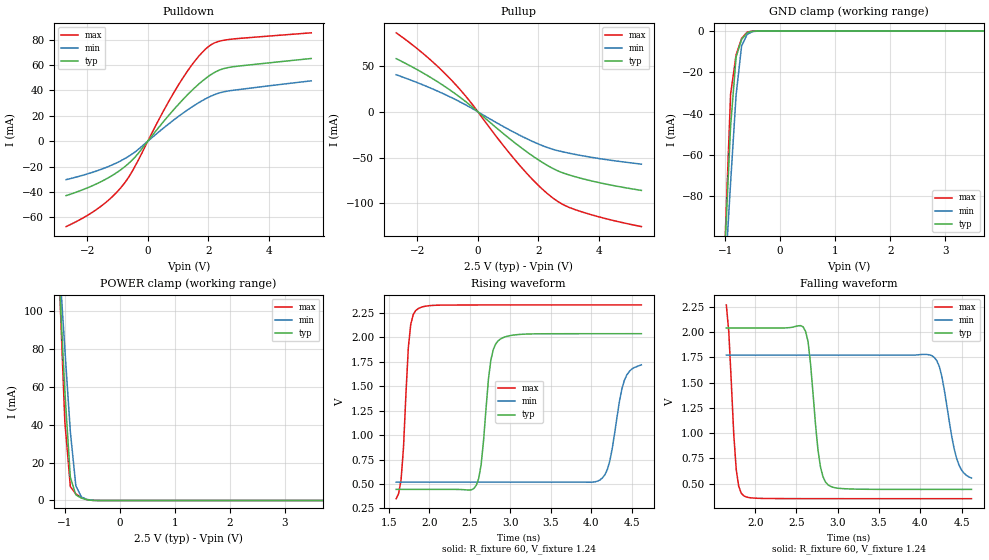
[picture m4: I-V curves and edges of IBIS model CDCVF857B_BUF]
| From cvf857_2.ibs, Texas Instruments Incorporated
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|   Diff. Driver Output  MODEL updated 8/2003
[Model]   CDCVF857B_BUF
Model_type   3-state
Polarity   Non-Inverting
| Signals   FBOUT,FBOUT-,Y0,Y0-, Y1,Y1-, Y2,Y2-, Y3,Y3-, Y4,Y4-,
|   Y5,Y5-, Y6,Y6-, Y7,Y7-, Y8,Y8-, Y9,Y9-
Vmeas = 1.25V   |Vref for timing measurements (crosspoint)
Cref = 14pF   |load capacitance for timing spec (to ground!)
Rref = 60   |60 Ohm to VDD/2 for timing measurements
Vref = 1.25V   |Timing specification test load voltage
| variable   typ   min   max
C_comp   2.4pF   2.0pF   2.7pF
[Temperature Range]   40.0   105   0
[Voltage range]   2.5V   2.3V   2.7V
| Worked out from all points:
|   slope of the pulldown table from 0 to 0.375 V, typ, clamps not added: 33.3 ohm
|   slope of the pullup table from 0 to 0.375 V, typ, clamps not added: 34.6 ohm
|   GND clamp passes 1 mA (typ) near -0.61 V on its own axis
|   POWER clamp passes 1 mA (typ) near -0.67 V on its own axis
|   rising waveform, R_fixture 60, V_fixture 1.24: 20-80 % time 105ps typ, 146ps min, 76.2ps max; typ from 0.444 V to 2.04 V
|   falling waveform, R_fixture 60, V_fixture 1.24: 20-80 % time 108ps typ, 157ps min, 74.9ps max; typ from 2.04 V to 0.445 V
[Pullup]
|   40C:2.5V:nominal 105C:2.3V:weak   0C:2.7V:strong
|   Voltage   I(typ)   I(min)   I(max)
-2.7V     58.06mA    40.49mA    86.29mA
-1.7V     40.25mA    27.85mA    60.54mA
-900mV    23.3mA     15.98mA    35.5mA
-300mV    8.384mA    5.704mA    12.94mA
700mV     -19.95mA   -13.47mA   -30.93mA
1.3V      -35.9mA    -24.18mA   -55.38mA
1.9V      -50.31mA   -33.72mA   -77.12mA
2.4V      -60.47mA   -40.15mA   -92.13mA
2.8V      -66.59mA   -43.63mA   -101mA
3.3V      -71.64mA   -47.04mA   -107.8mA
4.2V      -78.68mA   -51.97mA   -116.4mA
5.4V      -85.8mA    -57.13mA   -125.3mA
[Pulldown]
|   40C:2.5V:nominal   105C:2.3V:weak   0C:2.7V:strong
|   Voltage   I(typ)   I(min)   I(max)
-2.7V     -42.96mA   -30.37mA   -67.38mA
-1.6V     -32.59mA   -22.72mA   -52.28mA
-1.2V     -27.42mA   -18.96mA   -44.42mA
-800mV    -20.89mA   -14.29mA   -34.01mA
-400mV    -12.02mA   -8.101mA   -18.78mA
500mV     14.9mA     9.979mA    23.08mA
1.1V      31.31mA    21.04mA    47.7mA
1.5V      41.03mA    27.64mA    61.59mA
2V        51.1mA     34.55mA    74.57mA
2.3V      55.4mA     37.56mA    78.41mA
2.7V      58.27mA    39.76mA    80.29mA
5.4V      65.21mA    47.59mA    85.47mA
[GND Clamp]
|   40C:2.5V:nominal  105C:2.3V:weak   0C:2.7V:strong
|  Voltage   I(typ)   I(min)   I(max)
-2.7V     -1.103A    -887.8mA   -1.395A
-1.1V     -162.1mA   -163.9mA   -171.8mA
-900mV    -46.23mA   -73.5mA    -30.7mA
-800mV    -12.6mA    -30.96mA   -11.52mA
-700mV    -4.108mA   -7.28mA    -3.616mA
-600mV    -807.7uA   -1.647mA   -496.6uA
-500mV    -81.09uA   -268.7uA   -30.08uA
-300mV    -219.6nA   -2.842uA   -15.58nA
5.4V      252.8pA    5.148nA    125.2pA
[POWER Clamp]
|   40C:2.5V:nominal   105C:2.3V:weak   0C:2.7V:strong
|  Voltage   I(typ)   I(min)   I(max)
-2.7V     1.057A     849.3mA    1.339A
-1.1V     116.1mA    125.3mA    115.7mA
-1V       57.76mA    80.13mA    41.69mA
-900mV    12.21mA    36.35mA    7.299mA
-800mV    2.976mA    7.713mA    3.48mA
-700mV    1.27mA     1.885mA    1.613mA
-600mV    407.8uA    568.5uA    461.4uA
-400mV    5.905uA    16.46uA    4.279uA
5.4V      0A         0A         0A
[ramp]
| variable   typ   min   max
dV/dt_r   0.9566/1.0240E-10   0.7468/1.5201E-10   1.1331/6.9055E-11
dV/dt_f   0.9566/1.0535E-10   0.7468/1.6224E-10   1.1331/6.9424E-11
[Rising Waveform]
R_fixture = 60
V_fixture = 1.24
V_fixture_min = 1.14
V_fixture_max = 1.39
|   NOTE: WARNINGS generated by Innoveda Visual IBIS Editor are a best
|   compromise for ramp resulution and TPD prepresentation within
|   the 100 data point limits.
|   If rise/fall time analysis is mor important then TPD, use the
|   PLL-TYPE model which has better timing resolution.
|   40C:2.5V:nominal  105C:2.3V:weak   0C:2.7V:strong
|   Time   V(typ)   V(min)   V(max)
1.59ns    443.9mV    518mV      348.7mV
1.65ns    443.9mV    518mV      541.5mV
1.77ns    443.9mV    518mV      2.135V
1.86ns    443.9mV    518mV      2.294V
2.58ns    487.3mV    518mV      2.332V
2.76ns    1.768V     518mV      2.332V
2.85ns    1.966V     518mV      2.332V
4.11ns    2.038V     541.6mV    2.333V
4.41ns    2.038V     1.56V      2.333V
4.62ns    2.038V     1.719V     2.333V
[Falling Waveform]
R_fixture = 60
V_fixture = 1.24
V_fixture_min = 1.14
V_fixture_max = 1.39
|   40C:2.5V:nominal   105C:2.3V:weak  0C:2.7V:strong
|   Time   V(typ)   V(min)   V(max)
1.65ns    2.039V     1.77V      2.267V
1.77ns    2.039V     1.77V      640.7mV
1.86ns    2.039V     1.77V      382.1mV
2.61ns    2.006V     1.77V      353.6mV
2.76ns    836.2mV    1.77V      353.5mV
2.88ns    491.1mV    1.77V      353.4mV
4.14ns    444.7mV    1.765V     353.1mV
4.26ns    444.7mV    1.563V     353.1mV
4.44ns    444.6mV    750.5mV    353mV
4.62ns    444.6mV    557.1mV    353mV
